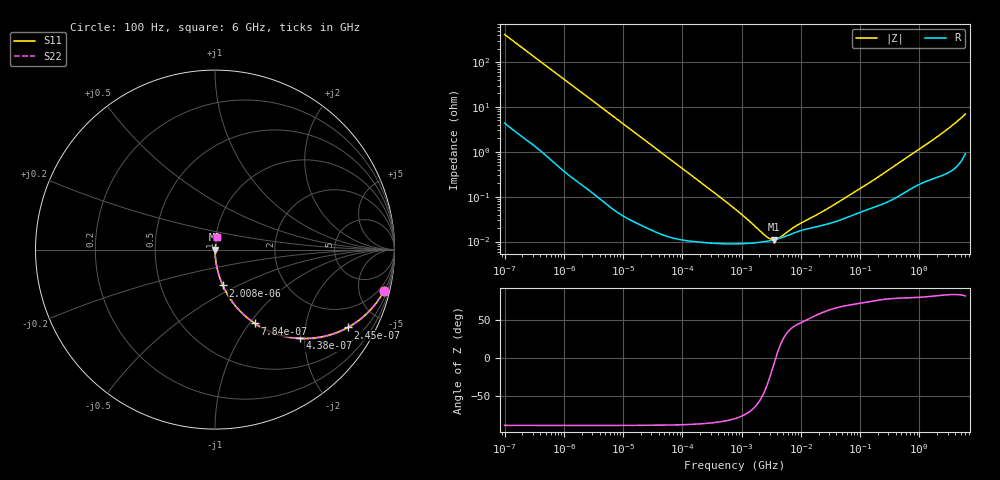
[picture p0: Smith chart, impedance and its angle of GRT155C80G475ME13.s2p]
!Murata Part Number: GRT155C80G475ME13
!These Parameters are Measured in Series Mode Connection
!Data Generated on Jun 19, 2026
!  o--ll--o
!Port1  Port2
!  o------o
!Operation Temp=25[degC], DC Bias Voltage=0[V]
!Freq. Start=100[Hz] Stop=6[GHz] 401[Steps]
# Hz S RI R 50
!Freq.(Hz) S11(Real) S11(Imag) S21(Real) S21(Imag) S12(Real) S12(Imag) S22(Real) S22(Imag)
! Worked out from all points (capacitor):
!   401 points, 100 Hz to 6 GHz, reference 50 ohm
!   read as one part in series: C = 3.85 uF near 109 Hz
!   lowest |Z| = 11 mohm at 3.55 MHz (marker M1)
!   series resonance near 3.767 MHz, so ESL is about 460 pH
!   S11 on the Smith chart (normalised r, x): 100 Hz: 1.09, -8.24; 245 Hz: 1.04, -3.38; 438 Hz: 1.02, -1.90; 784 Hz: 1.01, -1.06; 2.008 kHz: 1.00, -0.42; 6 GHz: 1.02, +0.14
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100  0.9422 -0.2281  0.0578 0.2281  0.0578 0.2281  0.9422 -0.2281
164  0.8619 -0.3399  0.1381 0.3399  0.1381 0.3399  0.8619 -0.3399
245  0.739 -0.434  0.261 0.434  0.261 0.434  0.739 -0.434
335  0.6048 -0.4837  0.3952 0.4837  0.3952 0.4837  0.6048 -0.4837
438  0.4744 -0.4943  0.5256 0.4943  0.5256 0.4943  0.4744 -0.4943
784  0.223 -0.4117  0.777 0.4117  0.777 0.4117  0.223 -0.4117
1227  0.1063 -0.3039  0.8937 0.3039  0.8937 0.3039  0.1063 -0.3039
2008  0.0434 -0.1995  0.9566 0.1995  0.9566 0.1995  0.0434 -0.1995
3437  0.0158 -0.1204  0.9842 0.1204  0.9842 0.1204  0.0158 -0.1204
6433  0.00483 -0.0653  0.9952 0.0653  0.9952 0.0653  0.00483 -0.0653
40335  0.000263 -0.0105  0.9997 0.0105  0.9997 0.0105  0.000263 -0.0105
774597  8.91e-05 -0.000527  0.9999 0.000527  0.9999 0.000527  8.91e-05 -0.000527
2594782  0.000101 -8.3e-05  0.9999 8.3e-05  0.9999 8.3e-05  0.000101 -8.3e-05
3103719  0.000106 -4.18e-05  0.9999 4.18e-05  0.9999 4.18e-05  0.000106 -4.18e-05
3549919  0.00011 -1.25e-05  0.9999 1.25e-05  0.9999 1.25e-05  0.00011 -1.25e-05
4440638  0.000119 3.42e-05  0.9999 -3.42e-05  0.9999 -3.42e-05  0.000119 3.42e-05
7947587  0.000159 0.000147  0.9998 -0.000147  0.9998 -0.000147  0.000159 0.000147
1.555665e7  0.000203 0.000283  0.9998 -0.000283  0.9998 -0.000283  0.000203 0.000283
9.326766e7  0.000435 0.00136  0.9996 -0.00136  0.9996 -0.00136  0.000435 0.00136
3.124326e8  0.000812 0.00397  0.9992 -0.00397  0.9992 -0.00397  0.000812 0.00397
1.95892e9  0.0031 0.0209  0.9969 -0.0209  0.9969 -0.0209  0.0031 0.0209
6e9  0.0137 0.0676  0.9863 -0.0676  0.9863 -0.0676  0.0137 0.0676
